| IBIS file rt600_fowlp249_dr2.ibs generated by Viper version: 2020.06.29
[IBIS Ver]   5.0
[Comment Char]   |_char
[File Name]   rt600_fowlp249_dr2.ibs
[File Rev]   1.3
[Date]   Mon Jun 29 17:46:21 2020
[Source]   NXP Viper 2020.06.29
[Notes]
[Disclaimer] IMPORTANT NOTICE
  This information is provided on an AS IS basis and without warranty.
  IN NO EVENT SHALL NXP BE LIABLE FOR INCIDENTAL OR CONSEQUENTIAL
  DAMAGES ARISING FROM USE OF THIS INFORMATION. THIS DISCLAIMER OF
  WARRANTY EXTENDS TO THE USER OF THE INFORMATION, AND TO THEIR CUSTOMERS
  OR USERS OF PRODUCTS  AND IS IN LIEU OF ALL WARRANTIES WHETHER EXPRESS,
  IMPLIED, OR STATUTORY, INCLUDING IMPLIED WARRANTIES OF MERCHANTABILITY
  OR FITNESS FOR PARTICULAR PURPOSE.
  NXP does not represent or warrant that the information furnished
  hereunder is free of infringement of any third party patents,
  copyrights, trade secrets, or other intellectual property rights.
  NXP does not represent or warrant that the information is free of
  defect, or that it meets any particular standard, requirements or need
  of the user of the infomation or their customers.
  NXP reserves the right to change the information in this file
  without notice.
   http://www.nxp.com
[Copyright]   (C) Copyright NXP 2004 - 2020, All Rights Reserved.
|   FOWLP249
[Component]   FOWLP249
[Manufacturer]   NXP
[Package]
| variable   typ   min   max
R_pkg   0.15685   0.025689   0.59036
L_pkg   1.022e-09   1.093e-10   3.895e-09
C_pkg   3.297e-13   1.257e-13   8.121e-13
[Pin] signal_name   model_name   R_pin   L_pin   C_pin
A1   GND   GND   NA   NA   NA
A2   XTALIN32KHZ   NC   0.31792   1.882e-09 2.750e-13
A4   XTALOUTSYS   NC   0.29043   1.430e-09 3.748e-13
A6   PIO0_28   gpio   0.23365   1.753e-09 2.937e-13
A8   PIO0_23   gpio   0.18331   1.237e-09 4.608e-13
A10   PIO0_22   gpio   0.14543   1.137e-09 3.823e-13
A12   PIO0_21   gpio   0.17444   1.307e-09 4.202e-13
A14   PIO0_18   gpio   0.28407   1.639e-09 5.811e-13
A16   PIO0_15   gpio   0.33013   1.989e-09 5.754e-13
A17   GND   GND   NA   NA   NA
B1   PIO0_31   gpio   0.52449   3.155e-09 5.133e-13
B2   VDD_AO18   POWER   NA   NA   NA
B3   XTALOUT32KHZ   NC   0.29778   1.834e-09 4.581e-13
B4   XTALINSYS   NC   0.27176   1.237e-09 5.171e-13
B6   PIO0_29   gpio   0.15495   1.310e-09 3.556e-13
B7   PIO0_25   gpio   0.18407   1.378e-09 2.558e-13
B8   PIO0_24   gpio   0.13563   1.129e-09 1.952e-13
B10   PIO3_9   gpio   0.09008   9.009e-10 3.412e-13
B11   PIO1_2   gpio   0.088334  8.545e-10 2.305e-13
B12   PIO0_16   gpio   0.11469   6.472e-10 3.785e-13
B14   PIO0_17   gpio   0.28166   1.570e-09 4.417e-13
B15   PIO1_8   gpio   0.25833   1.706e-09 2.958e-13
B16   PIO0_26   gpio   0.31195   1.903e-09 4.581e-13
B17   PIO0_14   gpio   0.33262   2.191e-09 5.445e-13
C2   PIO3_20   gpio   0.50853   3.216e-09 7.108e-13
C3   GND   GND   NA   NA   NA
C4   RESETN   gpio   0.043614  5.746e-10 2.493e-13
C5   LDO_ENABLE   gpio   0.029603  3.386e-10 2.091e-13
C6   PIO0_30   gpio   0.13446   1.317e-09 3.188e-13
C7   GND   GND   NA   NA   NA
C8   PIO3_12   gpio   0.050796  5.303e-10 1.734e-13
C9   PIO3_10   gpio   0.082374  6.288e-10 2.204e-13
C10   PIO3_8   gpio   0.053736  4.970e-10 1.998e-13
C11   GND   GND   NA   NA   NA
C12   PIO2_31   gpio   0.069906  7.200e-10 1.853e-13
C13   PIO3_6   gpio   0.090424  7.168e-10 1.466e-13
C14   PIO3_5   gpio   0.12805   1.032e-09 1.675e-13
C15   GND   GND   NA   NA   NA
C16   PIO3_4   gpio   0.25448   1.490e-09 4.001e-13
D1   PIO3_18   gpio   0.59036   3.895e-09 7.837e-13
D2   PIO3_19   gpio   0.58157   3.751e-09 8.121e-13
D3   PMIC_MODE0   reset   0.067338  7.186e-10 3.021e-13
D4   VDDEAO   POWER   NA   NA   NA
D5   PIO3_13   gpio   0.10944   6.658e-10 2.970e-13
D6   PIO3_22   gpio   0.054599  4.064e-10 1.305e-13
D7   GND   GND   NA   NA   NA
D8   PIO3_21   gpio   0.052921  4.292e-10 1.310e-13
D9   PIO3_11   gpio   0.025689  1.093e-10 1.657e-13
D10   PIO3_14   gpio   0.028169  1.162e-10 1.666e-13
D11   VSS_ADC_ANA   GND   NA   NA   NA
D12   PIO0_19   gpio   0.042162  1.505e-10 1.806e-13
D13   PIO0_27   gpio   0.031804  1.884e-10 1.751e-13
D14   PIO3_0   gpio   0.037745  3.566e-10 1.260e-13
D15   PIO3_1   gpio   0.1178   8.822e-10 3.796e-13
D16   PIO3_2   gpio   0.19242   1.229e-09 4.609e-13
D17   PIO3_3   gpio   0.26926   1.576e-09 5.280e-13
E3   PIO1_7   gpio   0.30241   2.158e-09 3.715e-13
E4   PMIC_MODE1   reset   0.041656  2.226e-10 2.005e-13
E5   PIO3_17   gpio   0.095943  5.736e-10 2.752e-13
E6   PIO3_16   gpio   0.14151   6.183e-10 3.744e-13
E7   GND   GND   NA   NA   NA
E8   VDD_PLL18   POWER   NA   NA   NA
E9   PIO3_15   gpio   0.062645  2.118e-10 2.260e-13
E10   PIO3_7   gpio   0.074605  2.636e-10 2.289e-13
E11   GND   GND   NA   NA   NA
E12   VDD33_ADC_ANA   POWER   NA   NA   NA
E13   PIO0_20   gpio   0.041331  2.401e-10 1.926e-13
E14   PIO1_9   gpio   0.04545   2.732e-10 2.255e-13
E15   PIO3_24   gpio   0.083893  6.882e-10 4.419e-13
F1   PIO2_25   gpio   0.32392   1.875e-09 6.076e-13
F2   PIO1_10   gpio   0.27522   1.727e-09 4.548e-13
F3   FC15_SDA   gpio   0.15372   9.562e-10 4.345e-13
F4   FC15_SCL   gpio   0.15797   9.880e-10 2.235e-13
F5   INTN   gpio   0.060258  2.422e-10 2.723e-13
F6   VDDE1   POWER   NA   NA   NA
F7   VDDE1   POWER   NA   NA   NA
F8   VDD_FUSE18   POWER   NA   NA   NA
F9   VDDE1   POWER   NA   NA   NA
F10   VDDE1   POWER   NA   NA   NA
F11   VDDE1   POWER   NA   NA   NA
F12   VREFH_ANA18   NC   NA   NA   NA
F13   PIO2_15   gpio   0.038135  1.682e-10 1.838e-13
F14   PIO2_14   gpio   0.030388  1.250e-10 1.725e-13
F15   PIO0_12   gpio   0.061477  4.741e-10 1.996e-13
F16   PIO0_5   gpio   0.10807   7.823e-10 3.693e-13
F17   PIO0_6   gpio   0.16315   9.630e-10 4.493e-13
G2   PIO2_24   gpio   0.24455   1.340e-09 3.402e-13
G3   GND   GND   NA   NA   NA
G4   GND   GND   NA   NA   NA
G5   GND   GND   NA   NA   NA
G6   VDD1V8   POWER   NA   NA   NA
G7   GND   GND   NA   NA   NA
G8   GND   GND   NA   NA   NA
G9   VDDCORE_CAP   POWER   NA   NA   NA
G10   GND   GND   NA   NA   NA
G11   GND   GND   NA   NA   NA
G12   VREFL_ANA   NC   NA   NA   NA
G13   GND   GND   NA   NA   NA
G14   GND   GND   NA   NA   NA
G15   GND   GND   NA   NA   NA
G16   PIO0_13   gpio   0.13169   4.184e-10 3.503e-13
H1   PIO2_27   gpio   0.22203   1.441e-09 5.041e-13
H2   PIO2_26   gpio   0.22119   1.391e-09 2.769e-13
H3   PIO1_4   gpio   0.093783  6.960e-10 3.018e-13
H4   PIO1_0   gpio   0.042016  1.257e-10 1.886e-13
H5   PIO1_1   gpio   0.048635  1.834e-10 1.992e-13
H6   VDD18_IOREF_1   POWER   NA   NA   NA
H7   VDD1V8_DRV   POWER   NA   NA   NA
H8   VDDCORE_CAP   POWER   NA   NA   NA
H9   VDDCORE_CAP   POWER   NA   NA   NA
H10   VDDCORE_CAP   POWER   NA   NA   NA
H11   GND   GND   NA   NA   NA
H12   PIO3_23   gpio   0.21129   5.714e-10 5.222e-13
H13   VDD18_ADC_ANA   POWER   NA   NA   NA
H14   PIO0_3   gpio   0.037251  1.187e-10 1.774e-13
H15   PIO0_2   gpio   0.04693   3.895e-10 2.318e-13
H16   PIO0_1   gpio   0.14397   5.554e-10 4.261e-13
H17   PIO0_0   gpio   0.18459   9.060e-10 4.377e-13
J3   PIO1_5   gpio   0.092732  7.078e-10 1.380e-13
J4   PIO1_3   gpio   0.081933  6.506e-10 1.602e-13
J5   VDDE1   POWER   NA   NA   NA
J6   VDDE1   POWER   NA   NA   NA
J7   VDD1V8_DRV   POWER   NA   NA   NA
J8   VDDCORE_CAP   POWER   NA   NA   NA
J9   VDDCORE_CAP   POWER   NA   NA   NA
J10   VDDCORE_CAP   POWER   NA   NA   NA
J11   VDDCORE_CAP   POWER   NA   NA   NA
J12   VDDE0   POWER   NA   NA   NA
J13   VDDE0   POWER   NA   NA   NA
J14   VDD18_IOREF_0   POWER   NA   NA   NA
J15   PIO0_7   gpio   0.080882  6.616e-10 2.028e-13
K1   PIO2_30   gpio   0.17841   1.343e-09 4.043e-13
K2   PIO2_28   gpio   0.15946   1.248e-09 2.596e-13
K3   PIO1_6   gpio   0.040103  3.145e-10 1.270e-13
K4   GND   GND   NA   NA   NA
K5   VDD_USB33   POWER   NA   NA   NA
K6   PIO2_1   sd_mmc   0.21165   5.570e-10 5.323e-13
K7   GND   GND   NA   NA   NA
K8   VDDCORE_CAP   POWER   NA   NA   NA
K9   VDDCORE_CAP   POWER   NA   NA   NA
K10   VDDCORE_CAP   POWER   NA   NA   NA
K11   GND   GND   NA   NA   NA
K12   VDDE0   POWER   NA   NA   NA
K13   PIO0_11   gpio   0.051177  1.769e-10 4.025e-13
K14   PIO1_11   gpio   0.038245  1.175e-10 1.835e-13
K15   PIO0_9   gpio   0.087066  7.473e-10 1.444e-13
K16   PIO0_8   gpio   0.10519   7.654e-10 3.026e-13
K17   PIO0_4   gpio   0.19002   1.095e-09 4.828e-13
L2   PIO2_29   gpio   0.11568   8.318e-10 2.617e-13
L3   GND   GND   NA   NA   NA
L4   GND   GND   NA   NA   NA
L5   GND   GND   NA   NA   NA
L6   GND   GND   NA   NA   NA
L7   GND   GND   NA   NA   NA
L8   GND   GND   NA   NA   NA
L9   VDDCORE_CAP   POWER   NA   NA   NA
L10   GND   GND   NA   NA   NA
L11   GND   GND   NA   NA   NA
L12   GND   GND   NA   NA   NA
L13   GND   GND   NA   NA   NA
L14   GND   GND   NA   NA   NA
L15   GND   GND   NA   NA   NA
L16   PIO0_10   gpio   0.16484   1.305e-09 2.357e-13
M1   PIO2_8   sd_mmc   0.22389   1.904e-09 4.844e-13
M2   PIO2_9   gpio   0.2007   1.607e-09 2.264e-13
M3   PIO2_10   gpio   0.10441   1.120e-09 2.239e-13
M4   PIO2_5   sd_mmc   0.083165  3.818e-10 2.470e-13
M5   PIO2_3   sd_mmc   0.11238   3.682e-10 2.773e-13
M6   VDD_USB18   POWER   NA   NA   NA
M7   VDDE2   POWER   NA   NA   NA
M8   VDDE2   POWER   NA   NA   NA
M9   VDDE0   POWER   NA   NA   NA
M10   VDDE0   POWER   NA   NA   NA
M11   GND   GND   NA   NA   NA
M12   VDDE0   POWER   NA   NA   NA
M13   PIO1_17   gpio   0.041043  1.582e-10 1.871e-13
M14   PIO1_14   gpio   0.16434   1.173e-09 1.804e-13
M15   PIO1_15   gpio   0.12167   7.010e-10 2.361e-13
M16   PIO1_13   gpio   0.17537   1.263e-09 3.763e-13
M17   PIO1_12   gpio   0.18915   1.382e-09 4.253e-13
N3   PIO2_11   gpio   0.069409  5.557e-10 3.862e-13
N4   PIO2_7   sd_mmc   0.054485  2.331e-10 2.039e-13
N5   PIO2_4   sd_mmc   0.048289  2.181e-10 1.976e-13
N6   PIO2_0   sd_mmc   0.045575  1.810e-10 1.936e-13
N7   GND   GND   NA   NA   NA
N8   PIO1_31   sd_mmc   0.054051  2.742e-10 2.037e-13
N9   PIO3_30   gpio   0.077769  2.522e-10 3.104e-13
N10   PIO7_28   gpio   0.063683  1.621e-10 2.711e-13
N11   GND   GND   NA   NA   NA
N12   PIO7_26   gpio   0.075522  3.027e-10 4.495e-13
N13   PIO2_20   gpio   0.044053  1.881e-10 3.981e-13
N14   PIO2_19   gpio   0.039096  1.692e-10 1.819e-13
N15   PIO2_13   gpio   0.08722   7.176e-10 2.188e-13
P1   PIO4_5   gpio   0.46749   3.191e-09 6.089e-13
P2   PIO4_6   gpio   0.42379   2.813e-09 6.725e-13
P3   PIO4_7   gpio   0.38593   2.538e-09 4.836e-13
P4   PIO2_6   sd_mmc   0.072297  6.023e-10 1.609e-13
P5   PIO1_30   sd_mmc   0.1285   1.021e-09 1.712e-13
P6   PIO2_2   sd_mmc   0.037019  1.785e-10 1.257e-13
P7   PIO3_31   gpio   0.033319  1.201e-10 1.766e-13
P8   PIO3_29   gpio   0.031269  1.293e-10 1.707e-13
P9   PIO3_26   gpio   0.039208  1.187e-10 1.807e-13
P10   PIO7_30   gpio   0.03109   1.403e-10 1.761e-13
P11   GND   GND   NA   NA   NA
P12   PIO7_25   gpio   0.059744  2.751e-10 2.215e-13
P13   PIO2_21   gpio   0.039499  2.046e-10 2.066e-13
P14   PIO2_22   gpio   0.034026  2.075e-10 1.882e-13
P15   PIO2_18   gpio   0.11456   9.164e-10 3.735e-13
P16   PIO2_16   gpio   0.16603   1.066e-09 4.198e-13
P17   PIO1_16   gpio   0.23741   1.229e-09 4.756e-13
R2   PIO4_4   gpio   0.42481   2.781e-09 6.329e-13
R3   GND   GND   NA   NA   NA
R4   PIO4_8   gpio   0.25573   1.804e-09 4.926e-13
R5   PIO4_9   gpio   0.19032   1.347e-09 4.042e-13
R6   PIO4_10   gpio   0.1198   8.849e-10 2.671e-13
R7   GND   GND   NA   NA   NA
R8   PIO3_28   gpio   0.062146  5.160e-10 2.083e-13
R9   PIO3_25   gpio   0.095607  6.349e-10 2.411e-13
R10   PIO7_29   gpio   0.067168  5.378e-10 2.122e-13
R11   GND   GND   NA   NA   NA
R12   PIO7_27   gpio   0.087407  8.625e-10 2.018e-13
R13   PIO4_0   gpio   0.036473  2.789e-10 1.761e-13
R14   PIO2_23   gpio   0.037747  3.969e-10 3.393e-13
R15   GND   GND   NA   NA   NA
R16   PIO2_17   gpio   0.18889   1.268e-09 4.589e-13
T1   USB0_DM   NC   0.50751   2.703e-09 6.205e-13
T2   USB0_VBUS_DETECT   NC   0.10237   1.519e-09 4.696e-13
T3   PIO4_3   gpio   0.38349   2.407e-09 5.297e-13
T4   PIO7_31   gpio   0.35373   2.476e-09 4.566e-13
T6   PIO1_28   sd_mmc   0.26603   2.118e-09 2.571e-13
T7   PIO1_27   sd_mmc   0.2423   1.946e-09 2.531e-13
T8   PIO3_27   gpio   0.10694   9.603e-10 2.984e-13
T10   PIO1_23   sd_mmc   0.13415   1.018e-09 1.648e-13
T11   PIO1_22   sd_mmc   0.093117  6.877e-10 3.629e-13
T12   PIO1_20   sd_mmc   0.10148   7.619e-10 3.309e-13
T14   PIO2_12   gpio   0.13723   8.241e-10 2.812e-13
T15   PIO7_24   gpio   0.19543   1.385e-09 3.894e-13
T16   PIO4_2   gpio   0.20555   1.472e-09 4.542e-13
T17   PIO4_1   gpio   0.25734   1.457e-09 5.382e-13
U1   GND   GND   NA   NA   NA
U2   USB0_DP   NC   0.49555   2.721e-09 6.162e-13
U4   PIO1_18   sd_mmc   0.35786   2.425e-09 5.901e-13
U6   PIO1_26   sd_mmc   0.27931   2.102e-09 3.972e-13
U8   PIO1_25   sd_mmc   0.18721   1.556e-09 1.909e-13
U10   PIO1_24   sd_mmc   0.13998   1.070e-09 4.172e-13
U12   PIO1_21   sd_mmc   0.14201   1.049e-09 4.082e-13
U14   PIO1_29   sd_mmc   0.1904   1.085e-09 4.636e-13
U16   PIO1_19   sd_mmc   0.29144   1.497e-09 6.039e-13
U17   GND   GND   NA   NA   NA
[Pin Mapping]   pulldown_ref   pullup_ref
A1   GND   NC
A2   NC   NC
A4   NC   NC
A6   GND   VDDE1
A8   GND   VDDE1
A10   GND   VDDE1
A12   GND   VDDE1
A14   GND   VDDE1
A16   GND   VDDE1
A17   GND   NC
B1   GND   VDDE1
B2   NC   VDD_AO18
B3   NC   NC
B4   NC   NC
B6   GND   VDDE1
B7   GND   VDDE1
B8   GND   VDDE1
B10   GND   VDDE1
B11   GND   VDDE1
B12   GND   VDDE1
B14   GND   VDDE1
B15   GND   VDDE1
B16   GND   VDDE1
B17   GND   VDDE1
C2   GND   VDDE1
C3   GND   NC
C4   GND   VDDEAO
C5   GND   VDDEAO
C6   GND   VDDE1
C7   GND   NC
C8   GND   VDDE1
C9   GND   VDDE1
C10   GND   VDDE1
C11   GND   NC
C12   GND   VDDE1
C13   GND   VDDE1
C14   GND   VDDE1
C15   GND   NC
C16   GND   VDDE1
D1   GND   VDDE1
D2   GND   VDDE1
D3   GND   VDDEAO
D4   NC   VDDEAO
D5   GND   VDDE1
D6   GND   VDDE1
D7   GND   NC
D8   GND   VDDE1
D9   GND   VDDE1
D10   GND   VDDE1
D11   VSS_ADC_ANA   NC
D12   GND   VDDE1
D13   GND   VDDE1
D14   GND   VDDE1
D15   GND   VDDE1
D16   GND   VDDE1
D17   GND   VDDE1
E3   GND   VDDE1
E4   GND   VDDEAO
E5   GND   VDDE1
E6   GND   VDDE1
E7   GND   NC
E8   NC   VDD_PLL18
E9   GND   VDDE1
E10   GND   VDDE1
E11   GND   NC
E12   NC   VDD33_ADC_ANA
E13   GND   VDDE1
E14   GND   VDDE1
E15   GND   VDDE1
F1   GND   VDDE1
F2   GND   VDDE1
F3   GND   VDDE1
F4   GND   VDDE1
F5   GND   VDDEAO
F6   NC   VDDE1
F7   NC   VDDE1
F8   NC   VDD_FUSE18
F9   NC   VDDE1
F10   NC   VDDE1
F11   NC   VDDE1
F12   NC   NC
F13   GND   VDDE0
F14   GND   VDDE0
F15   GND   VDDE0
F16   GND   VDDE0
F17   GND   VDDE0
G2   GND   VDDE1
G3   GND   NC
G4   GND   NC
G5   GND   NC
G6   NC   VDD1V8
G7   GND   NC
G8   GND   NC
G9   NC   VDDCORE_CAP
G10   GND   NC
G11   GND   NC
G12   NC   NC
G13   GND   NC
G14   GND   NC
G15   GND   NC
G16   GND   VDDE0
H1   GND   VDDE1
H2   GND   VDDE1
H3   GND   VDDE1
H4   GND   VDDE1
H5   GND   VDDE1
H6   NC   VDD18_IOREF_1
H7   NC   VDD1V8_DRV
H8   NC   VDDCORE_CAP
H9   NC   VDDCORE_CAP
H10   NC   VDDCORE_CAP
H11   GND   NC
H12   GND   VDDE1
H13   NC   VDD18_ADC_ANA
H14   GND   VDDE0
H15   GND   VDDE0
H16   GND   VDDE0
H17   GND   VDDE0
J3   GND   VDDE1
J4   GND   VDDE1
J5   NC   VDDE1
J6   NC   VDDE1
J7   NC   VDD1V8_DRV
J8   NC   VDDCORE_CAP
J9   NC   VDDCORE_CAP
J10   NC   VDDCORE_CAP
J11   NC   VDDCORE_CAP
J12   NC   VDDE0
J13   NC   VDDE0
J14   NC   VDD18_IOREF_0
J15   GND   VDDE0
K1   GND   VDDE1
K2   GND   VDDE1
K3   GND   VDDE1
K4   GND   NC
K5   NC   VDD_USB33
K6   GND   VDDE2
K7   GND   NC
K8   NC   VDDCORE_CAP
K9   NC   VDDCORE_CAP
K10   NC   VDDCORE_CAP
K11   GND   NC
K12   NC   VDDE0
K13   GND   VDDE0
K14   GND   VDDE0
K15   GND   VDDE0
K16   GND   VDDE0
K17   GND   VDDE0
L2   GND   VDDE1
L3   GND   NC
L4   GND   NC
L5   GND   NC
L6   GND   NC
L7   GND   NC
L8   GND   NC
L9   NC   VDDCORE_CAP
L10   GND   NC
L11   GND   NC
L12   GND   NC
L13   GND   NC
L14   GND   NC
L15   GND   NC
L16   GND   VDDE0
M1   GND   VDDE2
M2   GND   VDDE2
M3   GND   VDDE2
M4   GND   VDDE2
M5   GND   VDDE2
M6   NC   VDD_USB18
M7   NC   VDDE2
M8   NC   VDDE2
M9   NC   VDDE0
M10   NC   VDDE0
M11   GND   NC
M12   NC   VDDE0
M13   GND   VDDE0
M14   GND   VDDE0
M15   GND   VDDE0
M16   GND   VDDE0
M17   GND   VDDE0
N3   GND   VDDE2
N4   GND   VDDE2
N5   GND   VDDE2
N6   GND   VDDE2
N7   GND   NC
N8   GND   VDDE2
N9   GND   VDDE0
N10   GND   VDDE0
N11   GND   NC
N12   GND   VDDE0
N13   GND   VDDE0
N14   GND   VDDE0
N15   GND   VDDE0
P1   GND   VDDE0
P2   GND   VDDE0
P3   GND   VDDE0
P4   GND   VDDE2
P5   GND   VDDE2
P6   GND   VDDE2
P7   GND   VDDE0
P8   GND   VDDE0
P9   GND   VDDE0
P10   GND   VDDE0
P11   GND   NC
P12   GND   VDDE0
P13   GND   VDDE0
P14   GND   VDDE0
P15   GND   VDDE0
P16   GND   VDDE0
P17   GND   VDDE0
R2   GND   VDDE0
R3   GND   NC
R4   GND   VDDE0
R5   GND   VDDE0
R6   GND   VDDE0
R7   GND   NC
R8   GND   VDDE0
R9   GND   VDDE0
R10   GND   VDDE0
R11   GND   NC
R12   GND   VDDE0
R13   GND   VDDE0
R14   GND   VDDE0
R15   GND   NC
R16   GND   VDDE0
T1   NC   NC
T2   NC   NC
T3   GND   VDDE0
T4   GND   VDDE0
T6   GND   VDDE0
T7   GND   VDDE0
T8   GND   VDDE0
T10   GND   VDDE0
T11   GND   VDDE0
T12   GND   VDDE0
T14   GND   VDDE0
T15   GND   VDDE0
T16   GND   VDDE0
T17   GND   VDDE0
U1   GND   NC
U2   NC   NC
U4   GND   VDDE0
U6   GND   VDDE0
U8   GND   VDDE0
U10   GND   VDDE0
U12   GND   VDDE0
U14   GND   VDDE0
U16   GND   VDDE0
U17   GND   NC
|*   Model Selector   *
[Model Selector] gpio
io_obe1dse0sre0   5mA current driving capability, without slew rate
io_obe1dse0sre1   5mA current driving capability, with slew rate
io_obe1dse1sre0   10mA current driving capability, without slew rate
io_obe1dse1sre1   10mA current driving capability, with slew rate
[Model Selector] reset
io_rst_obe1dse0sre0   5mA current driving capability, without slew rate
io_rst_obe1dse0sre1   5mA current driving capability, with slew rate
io_rst_obe1dse1sre0   10mA current driving capability, without slew rate
io_rst_obe1dse1sre1   10mA current driving capability, with slew rate
[Model Selector] sd_mmc
BDPROGSCARUDQP_SDMMC_3V3SF_00_SD   PSW=0 PDRV=0 MODE=1V8 SD
BDPROGSCARUDQP_SDMMC_3V3SF_01_SD   PSW=0 PDRV=1 MODE=1V8 SD
BDPROGSCARUDQP_SDMMC_3V3SF_00_MMC   PSW=0 PDRV=0 MODE=1V8 MMC
BDPROGSCARUDQP_SDMMC_3V3SF_01_MMC   PSW=0 PDRV=1 MODE=1V8 MMC
BDPROGSCARUDQP_SDMMC_3V3SF_10   PSW=1 PDRV=0 MODE=3V3 SD & 3V3 MMC
BDPROGSCARUDQP_SDMMC_3V3SF_11   PSW=1 PDRV=1 MODE=3V3 SD & 3V3 MMC
BDPROGSCARUDQP_SDMMC_3V3SF_11_2v7   PSW=1 PDRV=1 MODE=2V7 SD & 2V7 MMC
BDPROGSCARUDQP_SDMMC_3V3SF_10_2v7   PSW=1 PDRV=0 MODE=2V7 SD & 2V7 MMC
| End [Component] FOWLP249
| Models and submodels in the file (16): BDPROGSCARUDQP_SDMMC_3V3SF_00_MMC (I/O), BDPROGSCARUDQP_SDMMC_3V3SF_00_SD (I/O), BDPROGSCARUDQP_SDMMC_3V3SF_01_MMC (I/O), BDPROGSCARUDQP_SDMMC_3V3SF_01_SD (I/O), BDPROGSCARUDQP_SDMMC_3V3SF_10 (I/O), BDPROGSCARUDQP_SDMMC_3V3SF_10_2v7 (I/O), BDPROGSCARUDQP_SDMMC_3V3SF_11 (I/O), BDPROGSCARUDQP_SDMMC_3V3SF_11_2v7 (I/O), io_obe1dse0sre0 (I/O), io_obe1dse0sre1 (I/O), io_obe1dse1sre0 (I/O), io_obe1dse1sre1 (I/O), io_rst_obe1dse0sre0 (I/O), io_rst_obe1dse0sre1 (I/O), io_rst_obe1dse1sre0 (I/O), io_rst_obe1dse1sre1 (I/O)
